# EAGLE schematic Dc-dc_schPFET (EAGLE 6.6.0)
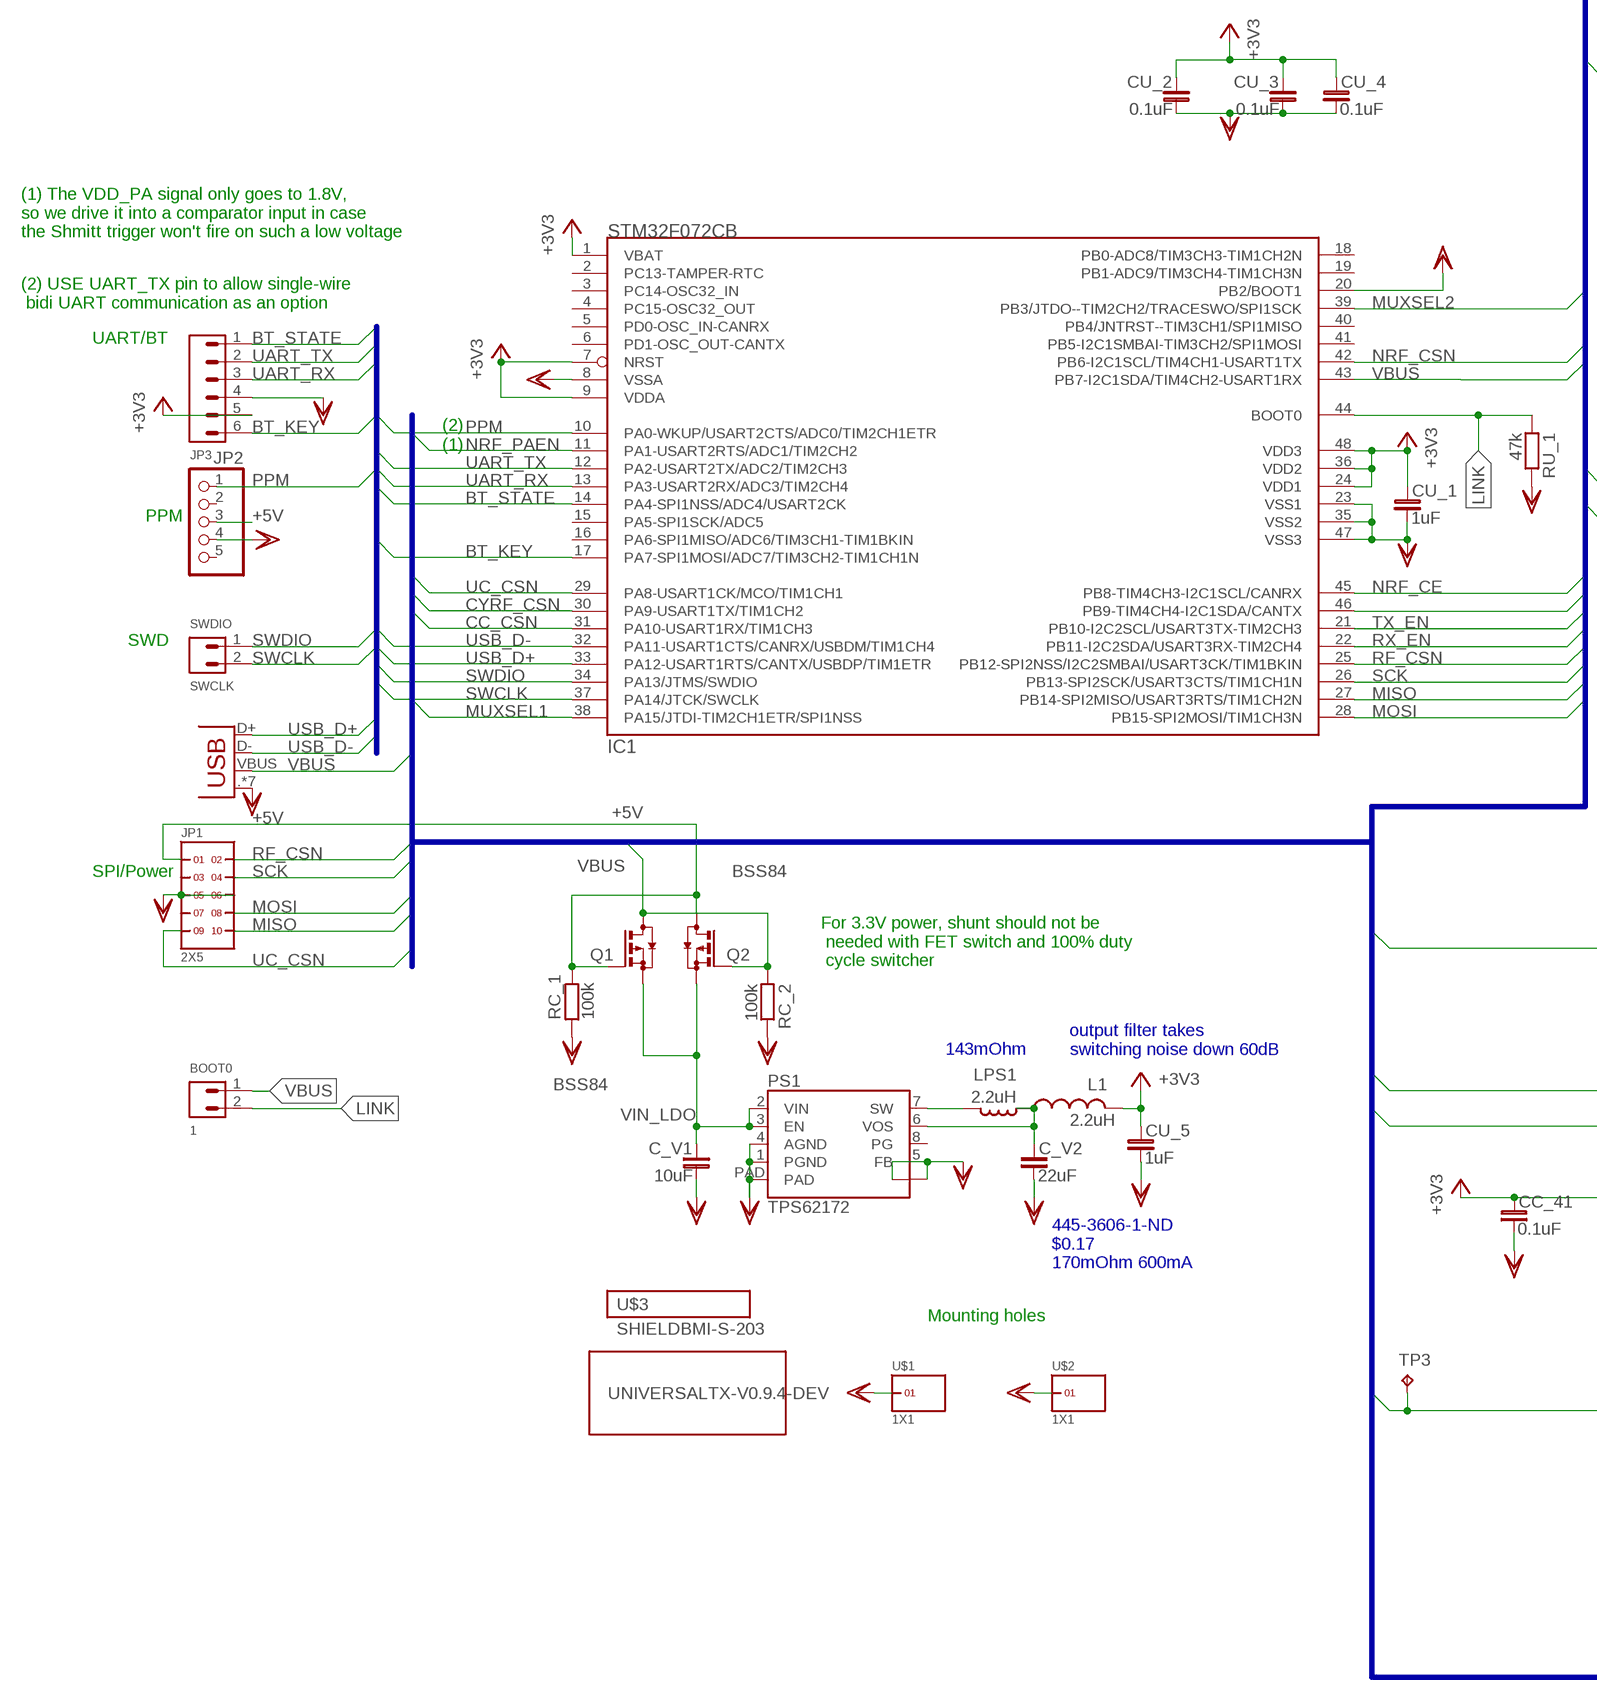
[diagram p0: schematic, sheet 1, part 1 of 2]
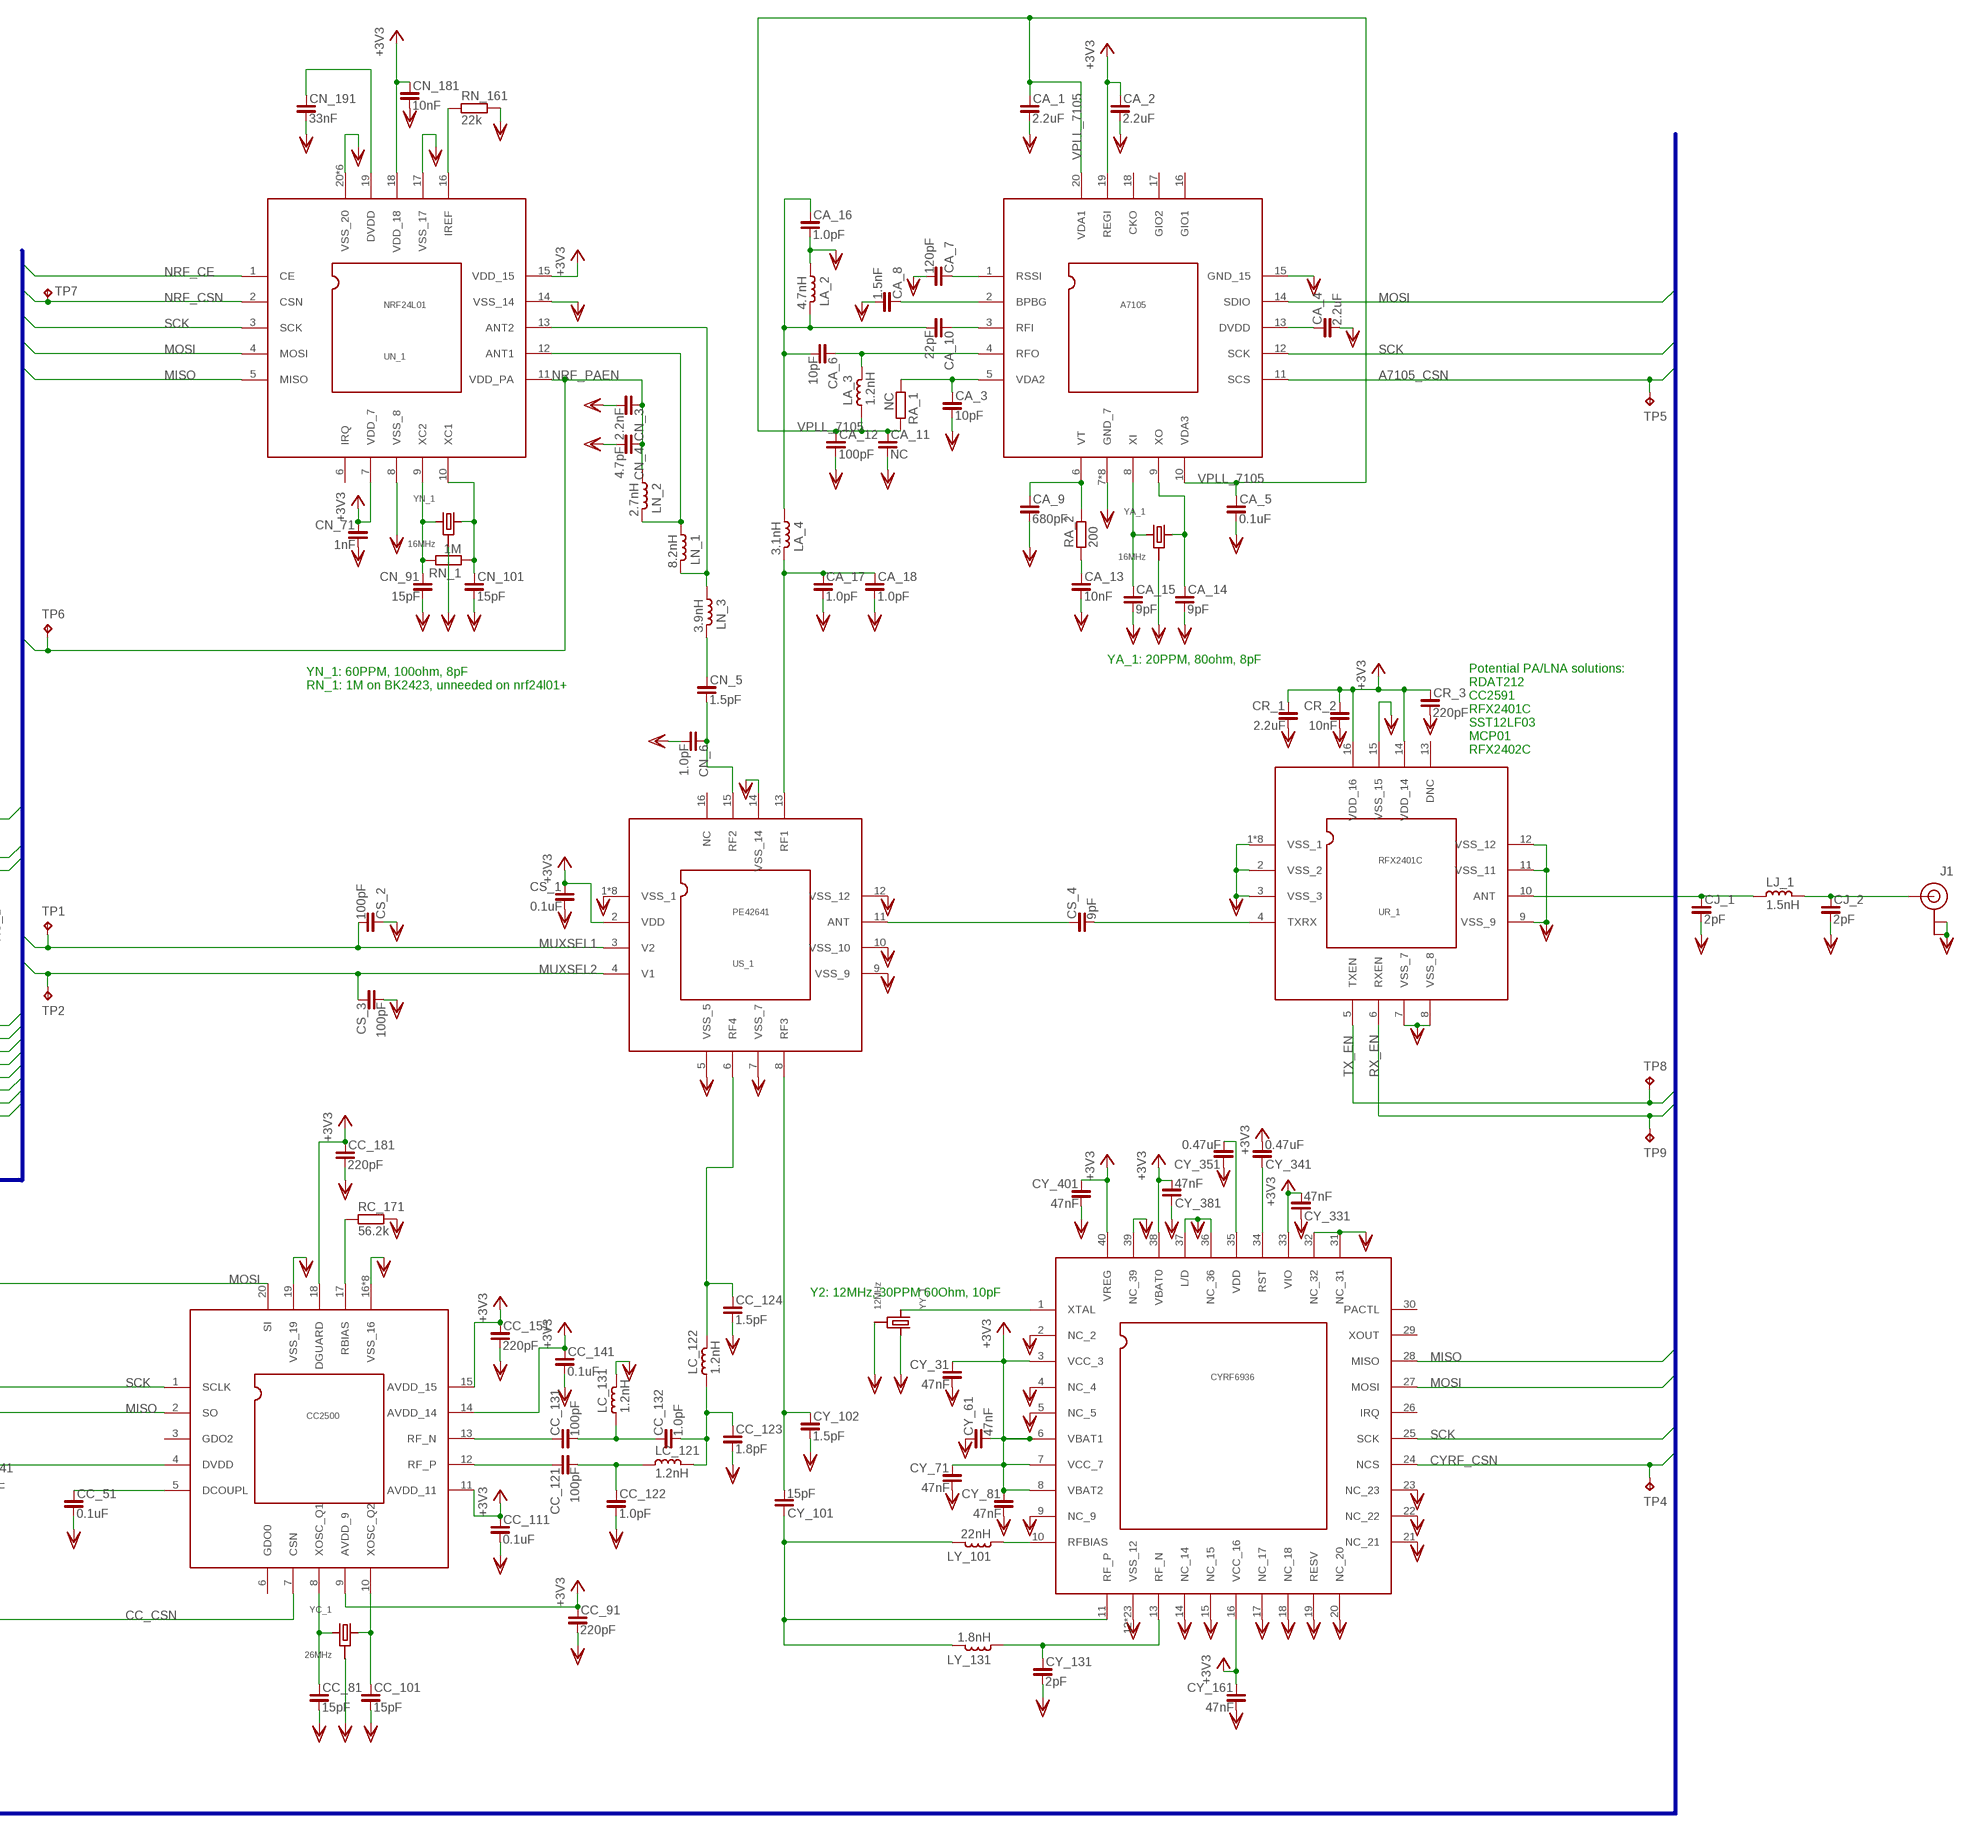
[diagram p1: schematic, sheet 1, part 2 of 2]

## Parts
1  BOOT0  PH1X2-05  [PH005-1-2]
C_V1  10uF  C_0805  [C0805]
C_V2  22uF  C_0805  [C0805]
CA_1  2.2uF  C_0402  [C0402]
CA_2  2.2uF  C_0402  [C0402]
CA_3  10pF  C_0402  [C0402]
CA_4  2.2uF  C_0402  [C0402]
CA_5  0.1uF  C_0402  [C0402]
CA_6  10pF  C_0402  [C0402]
CA_7  120pF  C_0402  [C0402]
CA_8  1.5nF  C_0402  [C0402]
CA_9  680pF  C_0402  [C0402]
CA_10  22pF  C_0402  [C0402]
CA_11  NC  C_0402  [C0402]
CA_12  100pF  C_0402  [C0402]
CA_13  10nF  C_0402  [C0402]
CA_14  9pF  C_0402  [C0402]
CA_15  9pF  C_0402  [C0402]
CA_16  1.0pF  C_0402  [C0402]
CA_17  1.0pF  C_0402  [C0402]
CA_18  1.0pF  C_0402  [C0402]
CC_41  0.1uF  C_0402  [C0402]
CC_51  0.1uF  C_0402  [C0402]
CC_81  15pF  C_0402  [C0402]
CC_91  220pF  C_0402  [C0402]
CC_101  15pF  C_0402  [C0402]
CC_111  0.1uF  C_0402  [C0402]
CC_121  100pF  C_0402  [C0402]
CC_122  1.0pF  C_0402  [C0402]
CC_123  1.8pF  C_0402  [C0402]
CC_124  1.5pF  C_0402  [C0402]
CC_131  100pF  C_0402  [C0402]
CC_132  1.0pF  C_0402  [C0402]
CC_141  0.1uF  C_0402  [C0402]
CC_151  220pF  C_0402  [C0402]
CC_181  220pF  C_0402  [C0402]
CJ_1  2pF  C_0402  [C0402]
CJ_2  2pF  C_0402  [C0402]
CN_3  2.2nF  C_0402  [C0402]
CN_4  4.7pF  C_0402  [C0402]
CN_5  1.5pF  C_0402  [C0402]
CN_6  1.0pF  C_0402  [C0402]
CN_71  1nF  C_0402  [C0402]
CN_91  15pF  C_0402  [C0402]
CN_101  15pF  C_0402  [C0402]
CN_181  10nF  C_0402  [C0402]
CN_191  33nF  C_0402  [C0402]
CR_1  2.2uF  C_0402  [C0402]
CR_2  10nF  C_0402  [C0402]
CR_3  220pF  C_0402  [C0402]
CS_1  0.1uF  C_0402  [C0402]
CS_2  100pF  C_0402  [C0402]
CS_3  100pF  C_0402  [C0402]
CS_4  9pF  C_0402  [C0402]
CU_1  1uF  C_0402  [C0402]
CU_2  0.1uF  C_0402  [C0402]
CU_3  0.1uF  C_0402  [C0402]
CU_4  0.1uF  C_0402  [C0402]
CU_5  1uF  C_0402  [C0402]
CY_31  47nF  C_0402  [C0402]
CY_61  47nF  C_0402  [C0402]
CY_71  47nF  C_0402  [C0402]
CY_81  47nF  C_0402  [C0402]
CY_101  15pF  C_0402  [C0402]
CY_102  1.5pF  C_0402  [C0402]
CY_131  2pF  C_0402  [C0402]
CY_161  47nF  C_0402  [C0402]
CY_331  47nF  C_0402  [C0402]
CY_341  0.47uF  C_0402  [C0402]
CY_351  0.47uF  C_0402  [C0402]
CY_381  47nF  C_0402  [C0402]
CY_401  47nF  C_0402  [C0402]
IC1  STM32F072CB  STM32-M-48  [LQFP48]
J1  U.FL  [U.FL]
JP1  2X5  [2X5]
JP2  PINHD-1X05_2.54-S  [1X05-S]
JP3  PH1X6-05  [PH005-1-6]
JP6  USBSMD  [USB-MINIB]
L1  2.2uH  INDUCTOR0603  [0603]
LA_2  4.7nH  L_0402  [L0402]
LA_3  1.2nH  L_0402  [L0402]
LA_4  3.1nH  L_0402  [L0402]
LC_121  1.2nH  L_0402  [L0402]
LC_122  1.2nH  L_0402  [L0402]
LC_131  1.2nH  L_0402  [L0402]
LJ_1  1.5nH  L_0402  [L0402]
LN_1  8.2nH  L_0402  [L0402]
LN_2  2.7nH  L_0402  [L0402]
LN_3  3.9nH  L_0402  [L0402]
LPS1  2.2uH  L_0805  [L0805]
LY_101  22nH  L_0402  [L0402]
LY_131  1.8nH  L_0402  [L0402]
PS1  TPS62172  [WSON-8-PAD]
Q1  BSS84  [SOT23]
Q2  BSS84  [SOT23]
RA_1  NC  R_0402  [R0402]
RA_2  200  R_0402  [R0402]
RC_1  100k  R_0402  [R0402]
RC_2  100k  R_0402  [R0402]
RC_171  56.2k  R_0402  [R0402]
RN_1  1M  R_0402  [R0402]
RN_161  22k  R_0402  [R0402]
RU_1  47k  R_0402  [R0402]
SWCLK  SWDIO  PH1X2-05  [PH005-1-2]
TP1  TPTP09R  [TP09R]
TP2  TPTP09R  [TP09R]
TP3  TPB1,27  [B1,27]
TP4  TPTP09R  [TP09R]
TP5  TPTP09R  [TP09R]
TP6  TPTP09R  [TP09R]
TP7  TPTP09R  [TP09R]
TP8  TPTP09R  [TP09R]
TP9  TPTP09R  [TP09R]
U$1  1X1  [1X1]
U$2  1X1  [1X1]
U$3  SHIELDBMI-S-203  [BMI-S-203-F]
UA_1  A7105  [A7105]
UC_1  CC2500  [CC2500]
UN_1  NRF24L01  [QFN20-4X4-NRF]
UNIVERSALTX-V0.9.4-DEV  LITTLE-GUYLITTLE-GUY-X  [LITTLE-GUY-X]
UR_1  RFX2401C  [QFN16-3X3-PAD]
US_1  PE42641  [QFN16-3X3-PAD]
UY_1  CYRF6936  [CYRF6936]
YA_1  16MHz  CRYSTAL.3.2X2.5MM  [3.2X2.5MM]
YC_1  26MHz  CRYSTAL.3.2X2.5MM  [3.2X2.5MM]
YN_1  16MHz  CRYSTAL.3.2X2.5MM  [3.2X2.5MM]
YY_1  12MHz  CRYSTAL.5X3.2MM  [5X3.2MM]

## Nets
+3V3: CA_2.1 CC_41.1 CC_91.1 CC_111.1 CC_141.1 CC_151.1 CC_181.1 CN_71.1 CN_181.1 CR_1.1 CR_2.1 CR_3.1 CS_1.1 CU_1.1 CU_2.1 CU_3.1 CU_4.1 CU_5.1 CY_31.1 CY_61.2 CY_71.1 CY_81.1 CY_161.1 CY_331.2 CY_341.2 CY_381.2 CY_401.1 IC1.1(VBAT) IC1.7(NRST) IC1.9(VDDA) IC1.24(VDD1) IC1.36(VDD2) IC1.48(VDD3) JP3.5 L1.2 UA_1.19(REGI) UC_1.4(DVDD) UC_1.9(AVDD_9) UC_1.11(AVDD_11) UC_1.14(AVDD_14) UC_1.15(AVDD_15) UC_1.18(DGUARD) UN_1.7(VDD_7) UN_1.15(VDD_15) UN_1.18(VDD_18) UR_1.14(VDD_14) UR_1.16(VDD_16) US_1.2(VDD) UY_1.3(VCC_3) UY_1.6(VBAT1) UY_1.7(VCC_7) UY_1.8(VBAT2) UY_1.16(VCC_16) UY_1.33(VIO) UY_1.38(VBAT0) UY_1.40(VREG)
+5V: JP1.1 JP2.3 Q1.1(G) Q2.3(D) RC_1.2
A7105_CSN: IC1.46(PB9-TIM4CH4-I2C1SDA/CANTX) TP5.TP UA_1.11(SCS)
BT_KEY: IC1.17(PA7-SPI1MOSI/ADC7/TIM3CH2-TIM1CH1N) JP3.6
BT_STATE: IC1.14(PA4-SPI1NSS/ADC4/USART2CK) JP3.1
CC_CSN: IC1.31(PA10-USART1RX/TIM1CH3) TP3.TP UC_1.7(CSN)
CYRF_CSN: IC1.30(PA9-USART1TX/TIM1CH2) TP4.TP UY_1.24(NCS)
LINK: 1.2 IC1.44(BOOT0) RU_1.1
MISO: IC1.27(PB14-SPI2MISO/USART3RTS/TIM1CH2N) JP1.10 UC_1.2(SO) UN_1.5(MISO) UY_1.28(MISO)
MOSI: IC1.28(PB15-SPI2MOSI/TIM1CH3N) JP1.8 UA_1.14(SDIO) UC_1.20(SI) UN_1.4(MOSI) UY_1.27(MOSI)
MUXSEL1: CS_2.2 IC1.38(PA15/JTDI-TIM2CH1ETR/SPI1NSS) TP1.TP US_1.3(V2)
MUXSEL2: CS_3.1 IC1.39(PB3/JTDO--TIM2CH2/TRACESWO/SPI1SCK) TP2.TP US_1.4(V1)
N$1: CN_101.1 RN_1.1 UN_1.10(XC1) YN_1.3
N$2: CN_91.1 RN_1.2 UN_1.9(XC2) YN_1.1
N$3: CN_191.1 UN_1.19(DVDD)
N$4: CA_9.1 RA_2.2 UA_1.6(VT)
N$5: LN_1.1 LN_3.2 UN_1.13(ANT2)
N$7: CJ_2.1 J1.P$3(SIGNAL) LJ_1.1
N$8: CN_5.1 LN_3.1
N$9: CN_5.2 CN_6.1 US_1.15(RF2)
N$10: RN_161.1 UN_1.16(IREF)
N$11: CA_13.1 RA_2.1
N$12: CA_14.1 UA_1.9(XO) YA_1.3
N$14: CC_131.1 UC_1.13(RF_N)
N$15: LN_1.2 LN_2.1 UN_1.12(ANT1)
N$16: CC_121.1 UC_1.12(RF_P)
N$17: CA_15.1 UA_1.8(XI) YA_1.1
N$18: CA_4.1 UA_1.13(DVDD)
N$24: CC_123.1 CC_132.2 LC_121.1 LC_122.2
N$25: CA_17.1 CA_18.1 LA_4.1 US_1.13(RF1)
N$26: CA_7.1 UA_1.1(RSSI)
N$27: CA_8.1 UA_1.2(BPBG)
N$28: CA_10.1 UA_1.3(RFI)
N$29: CA_6.1 LA_3.1 UA_1.4(RFO)
N$30: CA_3.1 RA_1.1 UA_1.5(VDA2)
N$31: CJ_1.1 LJ_1.2 UR_1.10(ANT)
N$32: CC_51.1 UC_1.5(DCOUPL)
N$33: CY_351.2 UY_1.35(VDD)
N$34: CS_4.1 US_1.11(ANT)
N$35: CS_4.2 UR_1.4(TXRX)
N$36: LPS1.1 PS1.7(SW)
N$37: RC_171.1 UC_1.17(RBIAS)
N$38: CC_101.1 UC_1.10(XOSC_Q2) YC_1.3
N$39: CC_81.1 UC_1.8(XOSC_Q1) YC_1.1
N$40: CC_121.2 CC_122.1 LC_121.2
N$41: CC_131.2 CC_132.1 LC_131.2
N$43: CY_341.1 UY_1.34(RST)
N$44: UY_1.1(XTAL) YY_1.1
N$45: LY_101.2 UY_1.10(RFBIAS)
N$46: CY_101.1 LY_101.1 LY_131.1 UY_1.11(RF_P)
N$47: CY_131.1 LY_131.2 UY_1.13(RF_N)
N$48: CA_6.2 CA_10.2 CA_16.1 LA_2.1 LA_4.2
N$49: CY_101.2 CY_102.1 US_1.8(RF3)
N$50: CC_124.1 LC_122.1 US_1.6(RF4)
N$51: C_V2.1 L1.1 LPS1.2 PS1.6(VOS)
NRF_CE: IC1.45(PB8-TIM4CH3-I2C1SCL/CANRX) UN_1.1(CE)
NRF_CSN: IC1.42(PB6-I2C1SCL/TIM4CH1-USART1TX) TP7.TP UN_1.2(CSN)
NRF_PAEN: CN_3.1 CN_4.1 IC1.11(PA1-USART2RTS/ADC1/TIM2CH2) LN_2.2 TP6.TP UN_1.11(VDD_PA)
PPM: IC1.10(PA0-WKUP/USART2CTS/ADC0/TIM2CH1ETR) JP2.1
RF_CSN: IC1.25(PB12-SPI2NSS/I2C2SMBAI/USART3CK/TIM1BKIN) JP1.2
RX_EN: IC1.22(PB11-I2C2SDA/USART3RX-TIM2CH4) TP9.TP UR_1.6(RXEN)
SCK: IC1.26(PB13-SPI2SCK/USART3CTS/TIM1CH1N) JP1.4 UA_1.12(SCK) UC_1.1(SCLK) UN_1.3(SCK) UY_1.25(SCK)
SWCLK: IC1.37(PA14/JTCK/SWCLK) SWCLK.2
SWDIO: IC1.34(PA13/JTMS/SWDIO) SWCLK.1
TX_EN: IC1.21(PB10-I2C2SCL/USART3TX-TIM2CH3) TP8.TP UR_1.5(TXEN)
UART_RX: IC1.13(PA3-USART2RX/ADC3/TIM2CH4) JP3.3
UART_TX: IC1.12(PA2-USART2TX/ADC2/TIM2CH3) JP3.2
UC_CSN: IC1.29(PA8-USART1CK/MCO/TIM1CH1) JP1.9
USB_D+: IC1.33(PA12-USART1RTS/CANTX/USBDP/TIM1ETR) JP6.D+
USB_D-: IC1.32(PA11-USART1CTS/CANRX/USBDM/TIM1CH4) JP6.D-
VBUS: 1.1 IC1.43(PB7-I2C1SDA/TIM4CH2-USART1RX) JP6.VBUS Q1.3(D) Q2.1(G) RC_2.1
VIN_LDO: C_V1.1 PS1.2(VIN) PS1.3(EN) Q1.2(S) Q2.2(S)
VPLL_7105: CA_1.1 CA_5.1 CA_11.1 CA_12.1 LA_3.2 RA_1.2 UA_1.10(VDA3) UA_1.20(VDA1)
VSS: C_V1.2 C_V2.2 CA_1.2 CA_2.2 CA_3.2 CA_4.2 CA_5.2 CA_7.2 CA_8.2 CA_9.2 CA_11.2 CA_12.2 CA_13.2 CA_14.2 CA_15.2 CA_16.2 CA_17.2 CA_18.2 CC_41.2 CC_51.2 CC_81.2 CC_91.2 CC_101.2 CC_111.2 CC_122.2 CC_123.2 CC_124.2 CC_141.2 CC_151.2 CC_181.2 CJ_1.2 CJ_2.2 CN_3.2 CN_4.2 CN_6.2 CN_71.2 CN_91.2 CN_101.2 CN_181.2 CN_191.2 CR_1.2 CR_2.2 CR_3.2 CS_1.2 CS_2.1 CS_3.2 CU_1.2 CU_2.2 CU_3.2 CU_4.2 CU_5.2 CY_31.2 CY_61.1 CY_71.2 CY_81.2 CY_102.2 CY_131.2 CY_161.2 CY_331.1 CY_351.1 CY_381.1 CY_401.2 IC1.8(VSSA) IC1.20(PB2/BOOT1) IC1.23(VSS1) IC1.35(VSS2) IC1.47(VSS3) J1.P$1(GND) J1.P$2(GND) JP1.5 JP1.6 JP2.4 JP3.4 JP6..(GND) JP6...(GND) JP6.GND JP6.MTN1(GND) JP6.MTN2(GND) JP6.MTN3(GND) JP6.MTN4(GND) LA_2.2 LC_131.1 PS1.1(PGND) PS1.4(AGND) PS1.5(FB) PS1.. PS1... PS1.PAD RC_1.1 RC_2.2 RC_171.2 RN_161.2 RU_1.2 U$1.2 U$2.2 UA_1.7(GND_7) UA_1.15(GND_15) UA_1.21(GND_7) UA_1.22(GND_7) UA_1.P$1(GND_7) UA_1.P$2(GND_7) UA_1.P$3(GND_7) UA_1.P$4(GND_7) UA_1.P$9(GND_7) UC_1.16(VSS_16) UC_1.19(VSS_19) UC_1.21(VSS_16) UC_1.22(VSS_16) UC_1.P$1(VSS_16) UC_1.P$2(VSS_16) UC_1.P$3(VSS_16) UC_1.P$4(VSS_16) UC_1.P$9(VSS_16) UN_1.8(VSS_8) UN_1.14(VSS_14) UN_1.17(VSS_17) UN_1.20(VSS_20) UN_1.P$1(VSS_20) UN_1.P$5(VSS_20) UN_1.P$6(VSS_20) UN_1.P$7(VSS_20) UN_1.P$9(VSS_20) UR_1.1(VSS_1) UR_1.2(VSS_2) UR_1.3(VSS_3) UR_1.7(VSS_7) UR_1.8(VSS_8) UR_1.9(VSS_9) UR_1.11(VSS_11) UR_1.12(VSS_12) UR_1.15(VSS_15) UR_1.17(VSS_1) UR_1.18(VSS_1) UR_1.P$1(VSS_1) UR_1.P$2(VSS_1) UR_1.P$3(VSS_1) UR_1.P$4(VSS_1) UR_1.P$5(VSS_1) US_1.1(VSS_1) US_1.5(VSS_5) US_1.7(VSS_7) US_1.9(VSS_9) US_1.10(VSS_10) US_1.12(VSS_12) US_1.14(VSS_14) US_1.17(VSS_1) US_1.18(VSS_1) US_1.P$1(VSS_1) US_1.P$2(VSS_1) US_1.P$3(VSS_1) US_1.P$4(VSS_1) US_1.P$5(VSS_1) UY_1.2(NC_2) UY_1.4(NC_4) UY_1.5(NC_5) UY_1.9(NC_9) UY_1.12(VSS_12) UY_1.14(NC_14) UY_1.15(NC_15) UY_1.17(NC_17) UY_1.18(NC_18) UY_1.19(RESV) UY_1.20(NC_20) UY_1.21(NC_21) UY_1.22(NC_22) UY_1.23(NC_23) UY_1.31(NC_31) UY_1.32(NC_32) UY_1.36(NC_36) UY_1.37(L/D) UY_1.39(NC_39) UY_1.P$1(VSS_12) UY_1.P$2(VSS_12) UY_1.P$3(VSS_12) UY_1.P$4(VSS_12) UY_1.P$5(VSS_12) UY_1.P$6(VSS_12) UY_1.P$7(VSS_12) UY_1.P$8(VSS_12) UY_1.P$9(VSS_12) UY_1.P$10(VSS_12) UY_1.P$11(VSS_12) UY_1.P$12(VSS_12) UY_1.P$13(VSS_12) UY_1.P$14(VSS_12) UY_1.P$15(VSS_12) UY_1.P$16(VSS_12) UY_1.P$17(VSS_12) UY_1.P$18(VSS_12) UY_1.P$19(VSS_12) UY_1.P$20(VSS_12) UY_1.P$21(VSS_12) UY_1.P$23(VSS_12) YA_1.2(VSS) YA_1.4(VSS) YC_1.2(VSS) YC_1.4(VSS) YN_1.2(VSS) YN_1.4(VSS) YY_1.2(VSS) YY_1.3 YY_1.4(VSS)
Unconnected: IC1.2(PC13-TAMPER-RTC) IC1.3(PC14-OSC32_IN) IC1.4(PC15-OSC32_OUT) IC1.5(PD0-OSC_IN-CANRX) IC1.6(PD1-OSC_OUT-CANTX) IC1.15(PA5-SPI1SCK/ADC5) IC1.16(PA6-SPI1MISO/ADC6/TIM3CH1-TIM1BKIN) IC1.18(PB0-ADC8/TIM3CH3-TIM1CH2N) IC1.19(PB1-ADC9/TIM3CH4-TIM1CH3N) IC1.40(PB4/JNTRST--TIM3CH1/SPI1MISO) IC1.41(PB5-I2C1SMBAI-TIM3CH2/SPI1MOSI) JP1.3 JP1.7 JP2.2 JP2.5 PS1.8(PG) UA_1.16(GIO1) UA_1.17(GIO2) UA_1.18(CKO) UC_1.3(GDO2) UC_1.6(GDO0) UN_1.6(IRQ) UR_1.13(DNC) US_1.16(NC) UY_1.26(IRQ) UY_1.29(XOUT) UY_1.30(PACTL)

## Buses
VBUS,SCK,MOSI,MISO,NRF_CSN,CC_CSN,A7105_CSN,CYRF_CSN,UC_CSN,RF_CSN,NRF_PAEN,MUXSEL1,MUXSEL2,TX_EN,RX_EN,NRF_CE
PPM,UART_TX,UART_RX,BT_KEY,BT_STATE,USB_D+,USB_D-,SWDIO,SWCLK,NRF_PAEN

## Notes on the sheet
- YA_1: 20PPM, 80ohm, 8pF
- YN_1: 60PPM, 100ohm, 8pF
  RN_1: 1M on BK2423, unneeded on nrf24l01+
- Potential PA/LNA solutions:
  RDAT212
  CC2591
  RFX2401C
  SST12LF03
  MCP01
  RFX2402C
- (1) The VDD_PA signal only goes to 1.8V,
  so we drive it into a comparator input in case
  the Shmitt trigger won't fire on such a low voltage
- (2) USE UART_TX pin to allow single-wire
   bidi UART communication as an option
- UART/BT
- (2)
- (1)
- PPM
- SWD
- SPI/Power
- For 3.3V power, shunt should not be
   needed with FET switch and 100% duty
   cycle switcher
- Y2: 12MHz, 30PPM 60Ohm, 10pF
- 143mOhm
- output filter takes 
  switching noise down 60dB
- 445-3606-1-ND 
  $0.17
  170mOhm 600mA
- Mounting holes

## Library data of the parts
1 SWCLK = UniversalTx:PH1X2
C_V1 C_V2 = rc-master-smd:C_: NON-POLARIZED CAP; DIGIKEY#: 490-1709-1-ND; MANF: Murata; MANF#: GRM21BR61A106KE19L; MOUSER#: 81-GRM21BR61A106KE19
CA_1 CA_2 CA_4 CR_1 = rc-master-smd:C_: NON-POLARIZED CAP; DIGIKEY#: 399-7375-1-ND; MANF: Kemet; MANF#: C0402C225M8PACTU; MOUSER#: 80-C0402C225M8P
CA_3 CA_6 = rc-master-smd:C_: NON-POLARIZED CAP; DIGIKEY#: 490-6186-1-ND; MANF: Murata; MANF#: GRM1555C1H100FA01D; MOUSER#: 81-GRM1555C1H100FA1D
CA_5 CC_41 CC_51 CC_111 CC_141 CS_1 CU_2-CU_4 = rc-master-smd:C_: NON-POLARIZED CAP; DIGIKEY#: 490-1318-1-ND; MANF: Murata; MANF#: GRM155R61A104KA01D; MOUSER#: 81-GRM155R61A104KA1D
CA_7 = rc-master-smd:C_: NON-POLARIZED CAP; DIGIKEY#: 490-8183-1-ND; MANF: Murata; MANF#: GRM1555C1H121GA01D; MOUSER#: 81-GRM1555C1H121GA1D
CA_8 = rc-master-smd:C_: NON-POLARIZED CAP; DIGIKEY#: 490-6354-1-ND; MANF: Murata; MANF#: GRM155R71H152KA01J; MOUSER#: 81-GRM155R71H152KA1J
CA_9 = rc-master-smd:C_: NON-POLARIZED CAP; DIGIKEY#: 490-3240-1-ND; MANF: Murata; MANF#: GRM1555C1H681JA01D; MOUSER#: 81-GRM1555C1H681JA1D
CA_10 = rc-master-smd:C_: NON-POLARIZED CAP; DIGIKEY#: 490-8173-1-ND; MANF: Murata; MANF#: GRM1555C1E220GA01D; MOUSER#: 81-GRM1555C1E220GA1D
CA_11 = rc-master-smd:C_: NON-POLARIZED CAP
CA_12 CC_121 CC_131 CS_2 CS_3 = rc-master-smd:C_: NON-POLARIZED CAP; DIGIKEY#: 490-6188-1-ND; MANF: Murata; MANF#: GRM1555C1H101GA01D; MOUSER#: 81-GRM1555C1H101GA1D
CA_13 CN_181 CR_2 = rc-master-smd:C_: NON-POLARIZED CAP; DIGIKEY#: 490-1313-1-ND; MANF: Murata; MANF#: GRM155R71C103KA01D; MOUSER#: 81-GRM155R71C103KA1D
CA_14 CA_15 CS_4 = rc-master-smd:C_: NON-POLARIZED CAP; DIGIKEY#: 490-6257-1-ND; MANF: Murata; MANF#: GRM1555C1H9R0BA01D; MOUSER#: 81-GRM1555C1H9R0BA1D
CA_16-CA_18 CC_122 CC_132 CN_6 = rc-master-smd:C_: NON-POLARIZED CAP; DIGIKEY#: 490-6206-1-ND; MANF: Murata; MANF#: GRM1555C1H1R0BA01D; MOUSER#: 81-GRM1555C1H1R0BA1D
CC_81 CC_101 CN_91 CN_101 CY_101 = rc-master-smd:C_: NON-POLARIZED CAP; DIGIKEY#: 490-6200-1-ND; MANF: Murata; MANF#: GRM1555C1H150FA01D; MOUSER#: 81-GRM1555C1H150FA1D
CC_91 CC_151 CC_181 CR_3 = rc-master-smd:C_: NON-POLARIZED CAP; DIGIKEY#: 490-1293-1-ND; MANF: Murata; MANF#: GRM1555C1H221JA01D; MOUSER#: 81-GRM1555C1H221JA1D
CC_123 = rc-master-smd:C_: NON-POLARIZED CAP; DIGIKEY#: 490-6215-1-ND; MANF: Murata; MANF#: GRM1555C1H1R8BA01D; MOUSER#: 81-GRM1555C1H1R8BA1D
CC_124 CN_5 CY_102 = rc-master-smd:C_: NON-POLARIZED CAP; DIGIKEY#: 490-6212-1-ND; MANF: Murata; MANF#: GRM1555C1H1R5BA01D; MOUSER#: 81-GRM1555C1H1R5BA1D
CJ_1 CJ_2 CY_131 = rc-master-smd:C_: NON-POLARIZED CAP; DIGIKEY#: 490-6226-1-ND; MANF: Murata; MANF#: GRM1555C1H2R0BA01D; MOUSER#: 81-GRM1555C1H2R0BA1D
CN_3 = rc-master-smd:C_: NON-POLARIZED CAP; DIGIKEY#: 490-6358-1-ND; MANF: Murata; MANF#: GRM155R71H222JA01D; MOUSER#: 81-GRM155R71H222JA1D
CN_4 = rc-master-smd:C_: NON-POLARIZED CAP; DIGIKEY#: 490-6244-1-ND; MANF: Murata; MANF#: GRM1555C1H4R7BA01D; MOUSER#: 81-GRM1555C1H4R7BA1D
CN_71 = rc-master-smd:C_: NON-POLARIZED CAP; DIGIKEY#: 490-3244-1-ND; MANF: Murata; MANF#: GRM1555C1H102JA01D; MOUSER#: 81-GRM1555C1H102JA1D
CN_191 = rc-master-smd:C_: NON-POLARIZED CAP; DIGIKEY#: 490-6333-1-ND; MANF: Murata; MANF#: GRM155R71C333KA01J; MOUSER#: 81-GRM155R71C333KA1J
CU_1 CU_5 = rc-master-smd:C_: NON-POLARIZED CAP; DIGIKEY#: 399-7766-1-ND; MANF: Kemet; MANF#: C0402C105M8PACTU; MOUSER#: 80-C0402C105M8P
CY_31 CY_61 CY_71 CY_81 CY_161 CY_331 CY_381 CY_401 = rc-master-smd:C_: NON-POLARIZED CAP; DIGIKEY#: 490-6473-1-ND; MANF: Murata; MANF#: GRM155R71C473KA01J; MOUSER#: 81-GRM155R71C473KA1J
CY_341 CY_351 = rc-master-smd:C_: NON-POLARIZED CAP; DIGIKEY#: 490-3266-1-ND; MANF: Murata; MANF#: GRM155R60J474KE19D; MOUSER#: 81-GRM155R60J474KE9D
IC1 = UniversalTx:STM32-M-48: STM32F103 Medium Density 48pins; DIGIKEY#: 497-14645-ND; MANF: STMicroelectronics; MANF#: STM32F072CBT6
J1 = UniversalTx:U.FL: SMD antenna connector- WRL-09144; DIGIKEY#: WM5587CT-ND; MANF: Molex; MANF#: 0734120110; PROD_ID: CONN-09193
JP1 = UniversalTx:2X5; DIGIKEY#: 952-1320-ND; MANF: Harwin; MANF#: M22-2520505
JP2 = UniversalTx:PINHD-1X05: PIN HEADER; DIGIKEY#: S7038-ND; MANF: Sullins; MANF#: PPPC051LFBN-RC
JP3 = UniversalTx:PH1X6
JP6 = UniversalTx:USB: USB Connectors USB-miniB is fully proven SKU : PRT-00587 USB-MICROB has been used. CONN-09505; DIGIKEY#: 670-1190-1-ND; MANF: JAE; MANF#: DX2R005HN2E700; PROD_ID: CONN-08193
L1 = SparkFun:INDUCTOR: Inductors
LA_2 = rc-master-smd:L_: INDUCTOR; DIGIKEY#: PCD1906CT-ND; MANF: Panasonic; MANF#: ELJ-RF4N7ZFB; MOUSER#: 667-ELJ-RF4N7ZFB
LA_3 LC_121 LC_122 LC_131 LPS1 = rc-master-smd:L_: INDUCTOR; DIGIKEY#: PCD1899CT-ND; MANF: Panasonic; MANF#: ELJ-RF1N2ZFB; MOUSER#: 667-ELJ-RF1N2ZFB
LA_4 = rc-master-smd:L_: INDUCTOR; DIGIKEY#: 535-10372-1-ND; MANF: Abracon; MANF#: ATFC-0402-3N1-BT
LJ_1 = rc-master-smd:L_: INDUCTOR; DIGIKEY#: PCD1900CT-ND; MANF: Panasonic; MANF#: ELJ-RF1N5ZFB; MOUSER#: 667-ELJ-RF1N5ZFB
LN_1 = rc-master-smd:L_: INDUCTOR; DIGIKEY#: PCD1909CT-ND; MANF: Panasonic; MANF#: ELJ-RF8N2ZFB; MOUSER#: 667-ELJ-RF8N2ZFB
LN_2 = rc-master-smd:L_: INDUCTOR; DIGIKEY#: PCD1903CT-ND; MANF: Panasonic; MANF#: ELJ-RF2N7ZFB; MOUSER#: 667-ELJ-RF2N7ZFB
LN_3 = rc-master-smd:L_: INDUCTOR; DIGIKEY#: PCD1905CT-ND; MANF: Panasonic; MANF#: ELJ-RF3N9ZFB; MOUSER#: 667-ELJ-RF3N9ZFB
LY_101 = rc-master-smd:L_: INDUCTOR; DIGIKEY#: PCD1914CT-ND; MANF: Panasonic; MANF#: ELJ-RF22NGFB; MOUSER#: 667-ELJ-RF22NGFB
LY_131 = rc-master-smd:L_: INDUCTOR; DIGIKEY#: PCD1901CT-ND; MANF: Panasonic; MANF#: ELJ-RF1N8ZFB; MOUSER#: 667-ELJ-RF1N8ZFB
PS1 = UniversalTx:TPS62172: Texas Instruments TPS62172 3-17V 0.5A Step-Down Converter with DCS control. Available in adjustable and fixed output voltage versions. Is packaged in an 8-pin WSON package measuring 2 Ã— 2 mm (DSG). See a 3.3V fixed output version of this chip in action on the Electric Imp Breakout Board. Datasheet; PROD_ID: IC-11307
Q1 Q2 = transistor-small-signal:BSS84: P-CHANNEL MOS FET
RA_1 = rc-master-smd:R_: RESISTOR
RA_2 = rc-master-smd:R_: RESISTOR; DIGIKEY#: P200JCT-ND; MANF: Panasonic; MANF#: ERJ-2GEJ201X; MOUSER#: 667-ERJ-2GEJ201X
RC_1 RC_2 RC_171 = rc-master-smd:R_: RESISTOR; DIGIKEY#: P56.2KLCT-ND; MANF: Panasonic; MANF#: ERJ-2RKF5622X; MOUSER#: 667-ERJ-2RKF5622X
RN_1 = rc-master-smd:R_: RESISTOR; DIGIKEY#: P1.0MJCT-ND; MANF: Panasonic; MANF#: ERJ-2GEJ105X; MOUSER#: 667-ERJ-2GEJ105X
RN_161 = rc-master-smd:R_: RESISTOR; DIGIKEY#: P22KJCT-ND; MANF: Panasonic; MANF#: ERJ-2GEJ223X; MOUSER#: 667-ERJ-2GEJ223X
RU_1 = rc-master-smd:R_: RESISTOR; DIGIKEY#: P10KJCT-ND; MANF: Panasonic; MANF#: ERJ-2GEJ103X; MOUSER#: 667-ERJ-2GEJ103X
TP1-TP9 = testpad:TP: Test pad
U$1 U$2 = UniversalTx:1X1
U$3 = UniversalTx:SHIELD
UA_1 = UniversalTx:A7105; MANF: Amiccom
UC_1 = UniversalTx:CC2500; DIGIKEY#: 296-19586-2-ND; MANF: TI; MANF#: CC2500RTKR
UN_1 = UniversalTx:NRF24L01: nRF24L01 Single chip 2.4GHz transceiver from Nordic Semiconductors.; DIGIKEY#: 1490-1033-1-ND; MANF: Nordic; MANF#: NRF24L01P-R7
UNIVERSALTX-V0.9.4-DEV = Deviation-Logos:LITTLE-GUY
UR_1 = UniversalTx:RFX2401C; MANF: RF Axis; MANF#: RFX2401C
US_1 = UniversalTx:PE42641
UY_1 = UniversalTx:CYRF6936; DIGIKEY#: 428-2962-ND; MANF: Cypress; MANF#: CYRF6936-40LTXC
YA_1 YN_1 = UniversalTx:CRYSTAL; DIGIKEY#: SER3628CT-ND; MANF: EPSON; MANF#: TSX-3225 16.0000MF09Z-AC3
YC_1 = UniversalTx:CRYSTAL; DIGIKEY#: 535-10916-1-ND; MANF: ABRACON; MANF#: ABM8G-26.000MHZ-4Y-T3
YY_1 = UniversalTx:CRYSTAL; DIGIKEY#: CTX833CT-ND; MANF: CTS; MANF#: 405C11A12M00000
